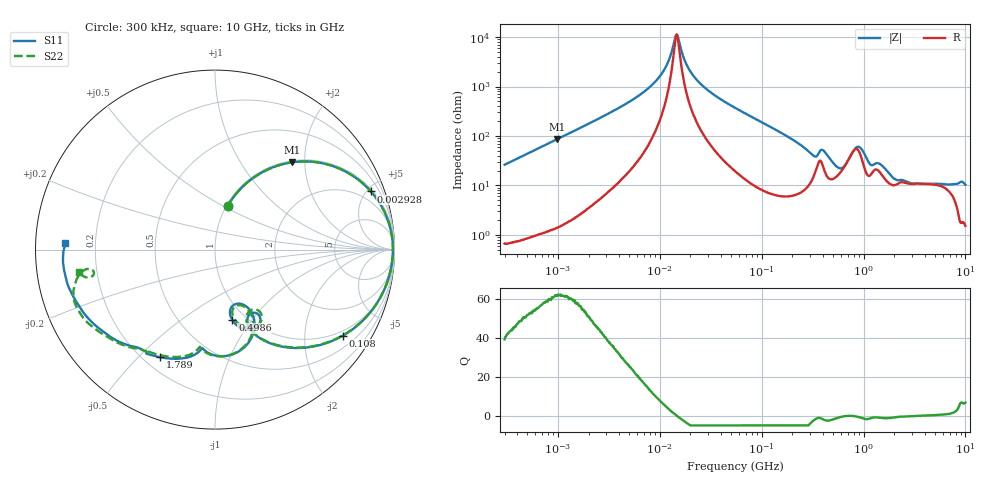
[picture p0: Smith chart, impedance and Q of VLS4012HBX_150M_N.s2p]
! S-Parameter Data Generated by TDK Corporation
! Copyright(C) 2023 TDK Corporation.
! All Rights Reserved.
! TDK P/N: VLS4012HBX-150M-N (Inductor)
! Property: L=15uH at 1MHz
! Size(LxWxT): 4x4x1.2mm
! Model Type: s2p (Touchstone File Format Version 1.0)
! Frequency: DC=Yes Start=0.3MHz Stop=10000MHz 802points Log-sweep
! Model Generated on June 16, 2023
! Port Assignments:
!  1 ---@@@--- 2
! Applicable Conditions:
!  Temperature = 25 degC
!  DC Bias Current = 0 A
!  Small Signal Operation
! Terms and conditions regarding TDK Simulation Models
! (1)This simulation model is being provided solely for informational purposes. Please refer to the specifications of the products in terms of detailed characteristics of such products.
! (2)In no event shall TDK Corporation of any of its subsidiaries be liable for any loss or damage arising, directly or indirectly,
!  From any information contained in this simulation model, including, but not limited to loss or damages arising from any inaccuracies, omissions or errors in connection with such information.
! (3)Any and all copyrights on this simulation model are owned by TDK Corporation.
!  Duplication or redistribution of this simulation model without prior written permission from TDK Corporation is prohibited.
! (4)This simulation model is subject to any modification or change without any prior notice.
! (5)Neither TDK Corporation nor any of its subsidiaries shall make any warranty, express or implied,
!  Including but not limited to the correctness, implied warranties of merchantability and fitness for a particular purpose with respect to this simulation models.
! (6)The use of this simulation model shall be deemed to have consented to the terms and conditions hereof.
# Hz S MA R 50
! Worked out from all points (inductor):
!   801 points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, 300 kHz to 10 GHz, reference 50 ohm
!   read as one part in series: L = 13.9 uH near 318.3 kHz
!   highest Q = 61.8 at 991.1 kHz (marker M1), where L = 13.9 uH
!   self-resonance near 14.54 MHz
!   S11 on the Smith chart (normalised r, x): 300 kHz: 1.01, +0.52; 2.928 MHz: 1.15, +5.30; 108 MHz: 0.84, -3.07; 498.6 MHz: 0.86, -0.81; 1.789 GHz: 0.27, -0.58; 10 GHz: 0.09, +0.02
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300000  0.2515 73.9  0.9614 -14.6  0.9614 -14.6  0.2515 73.9
991138  0.6497 48.5  0.7497 -40.6  0.7498 -40.6  0.6497 48.5
1713600  0.8262 33.2  0.5483 -55.8  0.5485 -55.8  0.8263 33.2
2927527  0.9273 20.4  0.3519 -68.1  0.352 -68.1  0.9274 20.5
9671944  0.9898 3.3  0.06722 -79.9  0.06728 -79.9  0.99 3.4
1.191229e7  0.9911 1.3  0.0337 -74.5  0.03371 -74.5  0.9912 1.3
1.470778e7  0.9911 -0.8  0.008785 1.1  0.008791 1.2  0.9913 -0.7
1.80882e7  0.9901 -2.8  0.03374 71.1  0.03375 71.2  0.9902 -2.7
2.252362e7  0.9877 -5.0  0.06839 76.6  0.06843 76.6  0.9878 -5.0
5.477226e7  0.9537 -17.5  0.2549 69.6  0.255 69.6  0.9539 -17.4
1.080141e8  0.8585 -34.0  0.4778 53.8  0.4779 53.7  0.8586 -33.7
1.923314e8  0.6807 -53.3  0.6912 33.3  0.6913 33.3  0.6805 -53.0
3.126428e8  0.4479 -66.1  0.7961 10.2  0.7963 10.2  0.4409 -66.4
3.860116e8  0.4801 -58.7  0.6925 6.1  0.6927 6.1  0.4665 -56.1
4.986356e8  0.4042 -76.2  0.8041 -1.0  0.8043 -1.0  0.408 -74.0
6.738867e8  0.3266 -67.1  0.7445 -17.7  0.7447 -17.7  0.3368 -66.7
8.528959e8  0.5008 -64.3  0.5723 -19.5  0.5724 -19.5  0.5026 -65.3
1.117505e9  0.574 -94.3  0.6891 -17.9  0.6893 -17.9  0.5723 -95.7
1.767019e9  0.6704 -116.3  0.626 -36.6  0.6261 -36.6  0.6648 -118.2
1.788985e9  0.6729 -117.0  0.6247 -37.2  0.6248 -37.2  0.6669 -118.9
4.22443e9  0.811 -154.0  0.3858 -75.4  0.386 -75.5  0.8094 -148.2
1e10  0.8368 177.6  0.2249 -111.2  0.2249 -111.3  0.7688 -170.8
